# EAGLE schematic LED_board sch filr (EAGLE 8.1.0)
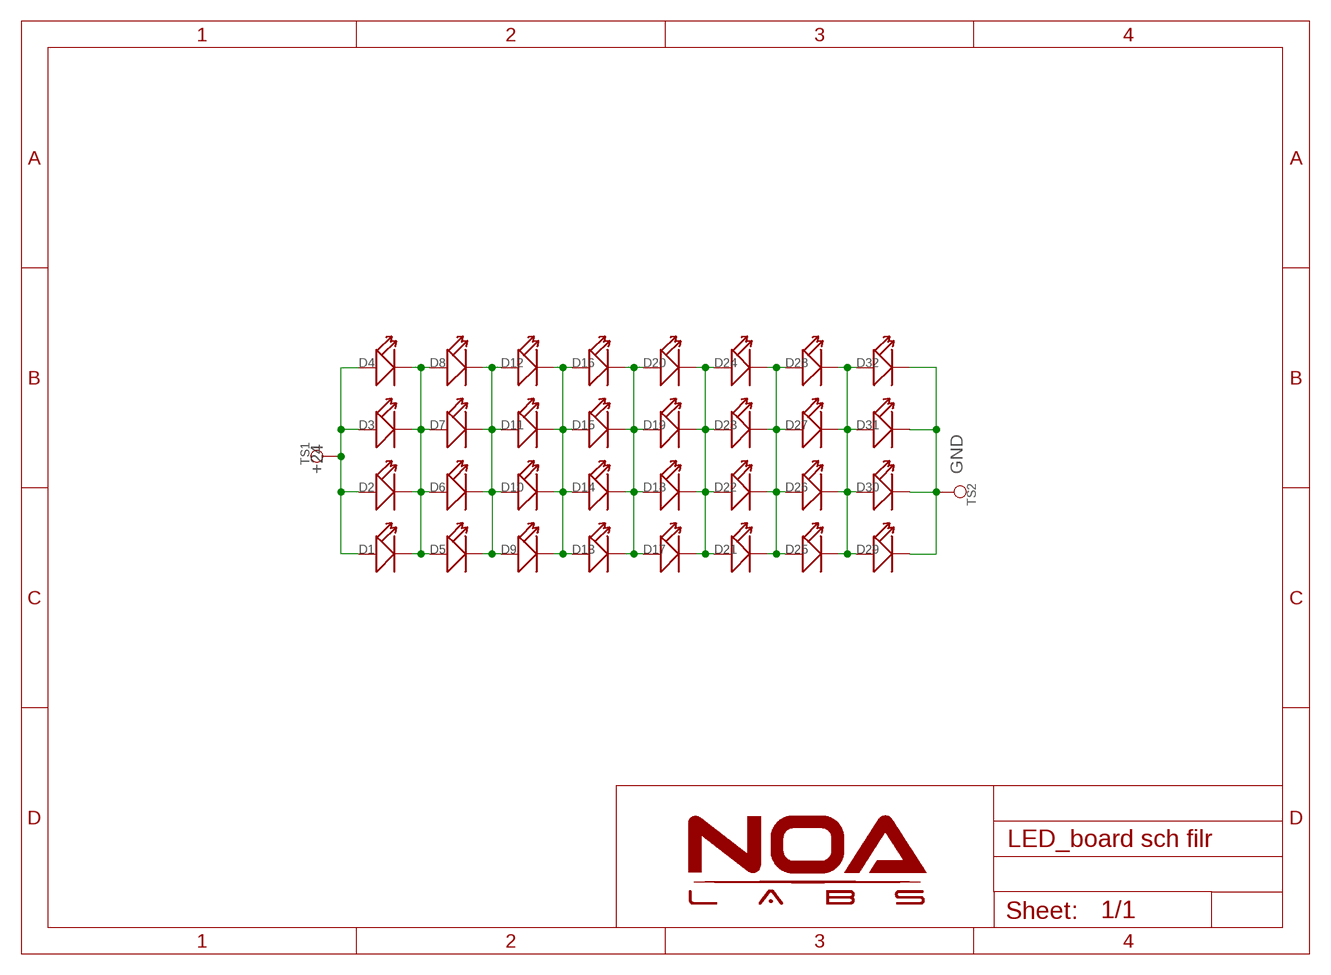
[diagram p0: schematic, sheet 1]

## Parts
D1  LED  [LED_2835]
D2  LED  [LED_2835]
D3  LED  [LED_2835]
D4  LED  [LED_2835]
D5  LED  [LED_2835]
D6  LED  [LED_2835]
D7  LED  [LED_2835]
D8  LED  [LED_2835]
D9  LED  [LED_2835]
D10  LED  [LED_2835]
D11  LED  [LED_2835]
D12  LED  [LED_2835]
D13  LED  [LED_2835]
D14  LED  [LED_2835]
D15  LED  [LED_2835]
D16  LED  [LED_2835]
D17  LED  [LED_2835]
D18  LED  [LED_2835]
D19  LED  [LED_2835]
D20  LED  [LED_2835]
D21  LED  [LED_2835]
D22  LED  [LED_2835]
D23  LED  [LED_2835]
D24  LED  [LED_2835]
D25  LED  [LED_2835]
D26  LED  [LED_2835]
D27  LED  [LED_2835]
D28  LED  [LED_2835]
D29  LED  [LED_2835]
D30  LED  [LED_2835]
D31  LED  [LED_2835]
D32  LED  [LED_2835]
TS1  TEST_POINT30MIL  [1P-30MIL]
TS2  TEST_POINT30MIL  [1P-30MIL]

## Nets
+24: D1.+ D2.+ D3.+ D4.+ TS1.P$1
GND: D29.- D30.- D31.- D32.- TS2.P$1
N$1: D1.- D2.- D3.- D4.- D5.+ D6.+ D7.+ D8.+
N$4: D5.- D6.- D7.- D8.- D9.+ D10.+ D11.+ D12.+
N$9: D9.- D10.- D11.- D12.- D13.+ D14.+ D15.+ D16.+
N$13: D13.- D14.- D15.- D16.- D17.+ D18.+ D19.+ D20.+
N$17: D17.- D18.- D19.- D20.- D21.+ D22.+ D23.+ D24.+
N$21: D21.- D22.- D23.- D24.- D25.+ D26.+ D27.+ D28.+
N$25: D25.- D26.- D27.- D28.- D29.+ D30.+ D31.+ D32.+

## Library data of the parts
D1-D32 = Discrete:LED*
TS1 TS2 = Connector:TEST_POINT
